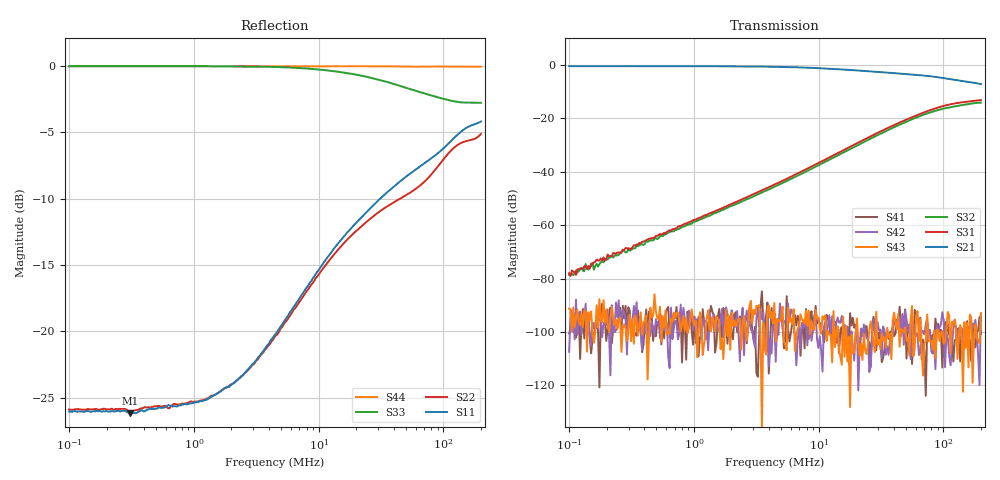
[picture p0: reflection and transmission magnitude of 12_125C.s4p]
!Keysight Technologies,E5080A,MY55200740,A.12.60.03
!Date: Friday, October 02, 2020 16:40:29
!Correction: S11(Full 4 Port(1,2,3,4))
!S12(Full 4 Port(1,2,3,4))
!S13(Full 4 Port(1,2,3,4))
!S14(Full 4 Port(1,2,3,4))
!S21(Full 4 Port(1,2,3,4))
!S22(Full 4 Port(1,2,3,4))
!S23(Full 4 Port(1,2,3,4))
!S24(Full 4 Port(1,2,3,4))
!S31(Full 4 Port(1,2,3,4))
!S32(Full 4 Port(1,2,3,4))
!S33(Full 4 Port(1,2,3,4))
!S34(Full 4 Port(1,2,3,4))
!S41(Full 4 Port(1,2,3,4))
!S42(Full 4 Port(1,2,3,4))
!S43(Full 4 Port(1,2,3,4))
!S44(Full 4 Port(1,2,3,4))
!S4P File: Measurements: <S11,S12,S13,S14>,
!<S21,S22,S23,S24>,
!<S31,S32,S33,S34>,
!<S41,S42,S43,S44>:Log Frequency Sweep
# Hz S  dB  R 50
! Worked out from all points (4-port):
!   300 points, 100 kHz to 200 MHz, reference 50 ohm
!   strongest paths, dB at 100 kHz, 673 kHz, 4.529 MHz, 30.48 MHz, 200 MHz:
!     S21: -0.5, -0.5, -0.7, -2.6, -7.2
!     S31: -78.0, -61.5, -44.5, -25.2, -13.1
!     S32: -78.6, -62.3, -45.3, -26.0, -14.1
!     S43: -91.3, -96.3, -103.7, -103.2, -92.9
!     S42: -107.4, -102.1, -111.2, -99.4, -93.5
!     S41: -100.6, -102.6, -104.2, -102.5, -100.8
!   lowest |S11| = -26.2 dB at 306 kHz (marker M1), VSWR 1.10, Z = 55.1 - j0.425 ohm
!   |S11| at or under -10 dB: start of sweep to 31.09 MHz
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100000  -26.05 0.1  -0.45 -0.2  -77.72 111.3  -86.42 89.0
        -0.45 -0.2  -25.89 0.3  -78.77 68.3  -89.02 -90.6
        -77.96 91.2  -78.59 97.7  0.00 -0.1  -90.62 1.9
        -100.55 -116.9  -107.40 -25.7  -91.29 -69.6  -0.00 -0.0
107924.7  -26.04 -0.1  -0.45 -0.2  -77.10 72.3  -90.39 -79.5
          -0.45 -0.2  -25.92 -0.3  -75.79 99.8  -87.08 75.9
          -77.41 90.0  -78.68 101.2  0.00 -0.2  -98.98 -75.7
          -99.93 -47.5  -92.79 120.5  -90.78 148.6  0.00 -0.0
306034.4  -26.18 -4.5  -0.45 -0.5  -68.30 91.0  -107.11 15.2
          -0.45 -0.4  -26.02 -3.8  -68.78 90.4  -95.56 -58.0
          -68.76 92.6  -69.52 90.4  -0.00 -0.4  -98.34 170.1
          -92.00 -65.5  -94.67 119.8  -93.46 -26.8  0.00 -0.0
2112653  -23.88 -49.3  -0.51 -2.7  -51.54 93.5  -101.31 39.2
         -0.51 -2.7  -23.87 -47.0  -52.32 93.6  -99.29 -0.8
         -51.57 92.9  -52.36 92.8  -0.02 -2.9  -97.74 46.5
         -93.62 -114.2  -98.23 51.1  -95.68 -51.2  -0.00 -0.2
1.928983e7  -11.98 -122.5  -1.97 -11.9  -29.83 94.4  -103.40 2.9
            -1.97 -11.9  -12.57 -112.5  -30.72 96.7  -103.31 119.5
            -29.82 94.4  -30.71 96.6  -0.61 -22.8  -96.63 -133.5
            -98.40 62.8  -110.69 -165.5  -107.52 17.8  -0.00 -1.3
8.215269e7  -6.88 -145.0  -4.32 -15.4  -16.58 58.8  -99.17 -100.1
            -4.33 -15.4  -8.04 -123.1  -17.47 67.5  -97.52 109.8
            -16.59 58.7  -17.46 67.5  -2.24 -68.4  -107.58 -53.4
            -101.02 69.4  -108.07 -159.5  -106.70 -42.9  -0.02 -5.7
2e8  -4.17 -157.3  -7.19 -10.3  -13.15 20.8  -101.43 107.6
     -7.19 -10.3  -5.11 -103.9  -14.10 44.4  -97.34 42.2
     -13.15 20.8  -14.10 44.4  -2.76 -112.7  -93.53 -109.7
     -100.77 -26.2  -93.52 119.0  -92.89 -143.1  -0.04 -13.4
